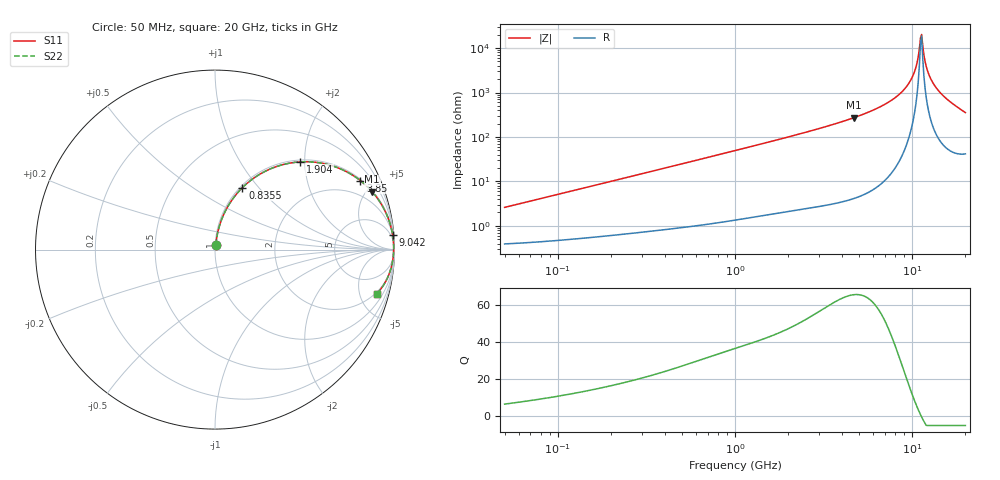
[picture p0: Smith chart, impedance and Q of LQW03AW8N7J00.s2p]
!Murata Part Number: LQW03AW8N7J00
!These Parameters are Measured in Series Mode Connection
!  o--[Z]--o
!Port1  Port2
!  o-------o
!Freq. Start=50[MHz] Stop=20[GHz], 401[Steps]
# Hz S RI R 50
!Freq.(Hz) S11(Real) S11(Imag) S21(Real) S21(Imag) S12(Real) S12(Imag) S22(Real) S22(Imag)
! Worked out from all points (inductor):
!   401 points, 50 MHz to 20 GHz, reference 50 ohm
!   read as one part in series: L = 8.17 nH near 51.52 MHz
!   highest Q = 65.8 at 4.678 GHz (marker M1), where L = 9.19 nH
!   self-resonance near 11.15 GHz
!   S11 on the Smith chart (normalised r, x): 50 MHz: 1.01, +0.05; 835.5 MHz: 1.02, +0.82; 1.904 GHz: 1.04, +1.90; 3.85 GHz: 1.07, +4.18; 9.042 GHz: 2, +24; 20 GHz: 1.83, -7.00
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5e7  0.00456 0.0255  0.9954 -0.0255  0.9954 -0.0255  0.00456 0.0255
1.364002e8  0.00987 0.068  0.9901 -0.068  0.9901 -0.068  0.00987 0.068
3.721004e8  0.0401 0.176  0.9599 -0.176  0.9599 -0.176  0.0401 0.176
8.354841e8  0.1523 0.345  0.8477 -0.345  0.8477 -0.345  0.1523 0.345
1e9  0.2021 0.3881  0.7979 -0.3881  0.7979 -0.3881  0.2021 0.3881
1.904239e9  0.4749 0.4887  0.5251 -0.4887  0.5251 -0.4887  0.4749 0.4887
2.728004e9  0.6584 0.4651  0.3416 -0.4651  0.3416 -0.4651  0.6584 0.4651
3.850025e9  0.8099 0.3845  0.1901 -0.3845  0.1901 -0.3845  0.8099 0.3845
4.677679e9  0.8757 0.3224  0.1243 -0.3224  0.1243 -0.3224  0.8757 0.3224
7.442007e9  0.9716 0.1556  0.0284 -0.1556  0.0284 -0.1556  0.9716 0.1556
9.041845e9  0.9895 0.0832  0.0105 -0.0832  0.0105 -0.0832  0.9895 0.0832
9.745021e9  0.9932 0.0551  0.00678 -0.0551  0.00678 -0.0551  0.9932 0.0551
1.019291e10  0.9946 0.0381  0.00537 -0.0381  0.00537 -0.0381  0.9946 0.0381
1.066139e10  0.9954 0.0211  0.0046 -0.0211  0.0046 -0.0211  0.9954 0.0211
1.098561e10  0.9956 0.00964  0.00443 -0.00964  0.00443 -0.00964  0.9956 0.00964
1.131968e10  0.9954 -0.00186  0.00457 0.00186  0.00457 0.00186  0.9954 -0.00186
1.149051e10  0.9953 -0.00763  0.00474 0.00763  0.00474 0.00763  0.9953 -0.00763
1.183995e10  0.9947 -0.0192  0.00533 0.0192  0.00533 0.0192  0.9947 -0.0192
1.220001e10  0.9938 -0.0309  0.00623 0.0309  0.00623 0.0309  0.9938 -0.0309
1.334722e10  0.989 -0.0666  0.011 0.0666  0.011 0.0666  0.989 -0.0666
1.573793e10  0.9704 -0.1351  0.0296 0.1351  0.0296 0.1351  0.9704 -0.1351
2e10  0.9006 -0.2457  0.0994 0.2457  0.0994 0.2457  0.9006 -0.2457
